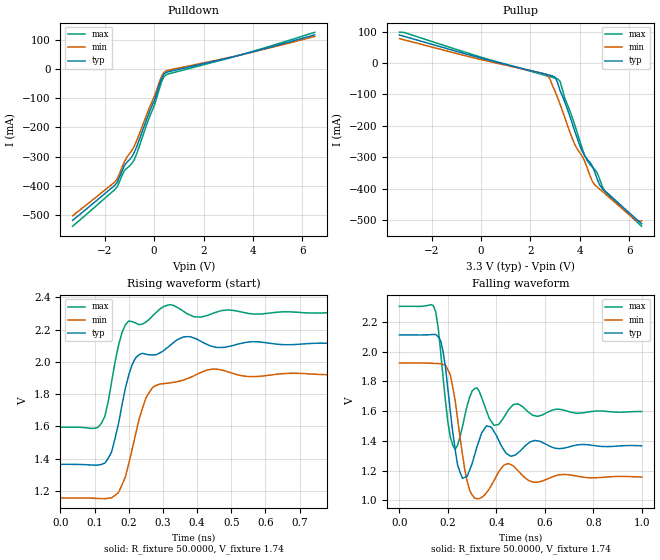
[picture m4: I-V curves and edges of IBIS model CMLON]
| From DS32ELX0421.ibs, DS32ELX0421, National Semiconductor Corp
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|   Model CMLON
[Model]  CMLON
Model_type Output
Polarity   Inverting
Vmeas =  1.792
Rref =   50.0000
Vref =   1.7415
C_comp   1.5000pF   NA   NA
[Temperature Range]   25.0000   85.0000   -40.0000
[Voltage Range]   3.3000V   3.000V   3.46500V
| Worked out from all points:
|   slope of the pulldown table from 0 to 0.495 V, typ, clamps not added: 5.02 ohm
|   slope of the pullup table from 0 to 0.495 V, typ, clamps not added: 49.3 ohm
|   rising waveform, R_fixture 50.0000, V_fixture 1.74: 20-80 % time 48.4ps typ, 56.4ps min, 39.9ps max; typ from 1.36 V to 2.11 V
|   falling waveform, R_fixture 50.0000, V_fixture 1.74: 20-80 % time 32.3ps typ, 41.2ps min, 25.8ps max; typ from 2.11 V to 1.37 V
[Pulldown]
|Voltage   I(typ)   I(min)   I(max)
-3.3V     -520.1mA   -504.3mA   -540.5mA
-1.6V     -400.1mA   -388.8mA   -414.9mA
-1.5V     -390mA     -377.8mA   -405.3mA
-1.2V     -331.2mA   -317.6mA   -348.3mA
-800mV    -285.5mA   -263.6mA   -310.2mA
-200mV    -148.9mA   -134.1mA   -166.4mA
1.971fV   -109mA     -94.64mA   -125.8mA
300mV     -31.75mA   -23.79mA   -42.53mA
400mV     -15.89mA   -9.943mA   -24.55mA
600mV     -7.505mA   -2.208mA   -15.04mA
3.4V      47.88mA    48.18mA    47.62mA
6.5V      119.3mA    113.5mA    128mA
[Pullup]
|Voltage   I(typ)   I(min)   I(max)
-3.3V     89.88mA    78.28mA    98.51mA
2.6V      -35mA      -34.6mA    -39.02mA
3V        -45.2mA    -90.63mA   -47.86mA
3.1V      -62.58mA   -110mA     -50.2mA
3.2V      -88.08mA   -131.3mA   -58.51mA
3.7V      -194mA     -241.7mA   -174.9mA
4.2V      -296.3mA   -314mA     -295.1mA
4.6V      -347mA     -388.2mA   -339mA
4.8V      -388.5mA   -401.7mA   -369.9mA
5V        -406.4mA   -415.4mA   -408.7mA
6.3V      -498.6mA   -503.7mA   -505.9mA
6.5V      -512.6mA   -503.7mA   -520.5mA
[Ramp]
| variable   typ   min   max
dV/dt_r   456.047m/53.64p   444.032m/59.22p   461.990m/48.80p
dV/dt_f   450.06m/35.89p   449.935m/41.09p   462.100m/35.41p
R_load = 50.00
[Rising Waveform]
R_fixture= 50.0000
V_fixture= 1.74
V_fixture_min= 1.54
V_fixture_max= 1.95
|time   V(typ)   V(min)   V(max)
0s        1.364V     1.155V     1.595V
120ps     1.364V     1.152V     1.619V
150ps     1.443V     1.157V     1.878V
170ps     1.618V     1.19V      2.102V
190ps     1.837V     1.287V     2.229V
220ps     2.024V     1.55V      2.241V
250ps     2.048V     1.775V     2.247V
310ps     2.083V     1.867V     2.349V
450ps     2.093V     1.955V     2.304V
1ns       2.113V     1.923V     2.306V
[Falling Waveform]
R_fixture= 50.0000
V_fixture= 1.74
V_fixture_min= 1.54
V_fixture_max= 1.95
|time   V(typ)   V(min)   V(max)
0s        2.113V     1.925V     2.305V
140ps     2.116V     1.922V     2.31V
180ps     2.003V     1.915V     1.832V
210ps     1.601V     1.844V     1.426V
230ps     1.343V     1.673V     1.343V
260ps     1.149V     1.313V     1.495V
310ps     1.304V     1.016V     1.751V
390ps     1.465V     1.132V     1.505V
460ps     1.297V     1.242V     1.627V
1ns       1.367V     1.158V     1.598V
